(* Logix 5000 AddOnInstructionDefinition export YAI_Assy_170_115_EIP_Hz; software revision 21.03 *)

ADD_ON_INSTRUCTION YAI_Assy_170_115_EIP_Hz   (* revision 1.0, vendor Yaskawa America, Inc. *)
// YAI Assembly 170 and 115
// Help:
// This add-on instruction is for use with input assemblie 166 and output assemblies 116.
// Node_Input_Assy is defined as the node's input assembly integer array.
// Node_Output_Assy is defined as the node's output assembly integer array.
// Torque limit/reference, torque compensation and torque output variables are only available with A1000.
VAR_IN_OUT
   Node_Input_Assy : AB:ETHERNET_MODULE_INT_24Bytes:I:0; {required}   // Input assembly words
   Node_Output_Assy : AB:ETHERNET_MODULE_INT_40Bytes:O:0; {required}   // Output assembly words
END_VAR
VAR_INPUT
   RunFwd : BOOL; {visible}   // Forward run command
   RunRev : BOOL; {visible}   // Reverse run command
   MFI_3 : BOOL; {visible}   // Multi-function input 3
   MFI_4 : BOOL; {visible}   // Multi-function input 4
   MFI_5 : BOOL; {visible}   // Multi-function input 5
   MFI_6 : BOOL; {visible}   // Multi-function input 6
   MFI_7 : BOOL; {visible}   // Multi-function input 7
   MFI_8 : BOOL; {visible}   // Multi-function input 8
   External_Fault : BOOL;   // External fault command (EF0)
   FaultReset : BOOL; {visible}   // Fault reset command
   MFO_1 : BOOL; {visible}   // Multi-function output (M1-M2 for A/P1000, MA/MB/MC for V1000)
   MFO_2 : BOOL; {visible}   // Multi-function output (M3-M4 for A/P1000, P1 for V1000)
   MFO_3 : BOOL; {visible}   // Multi-function output (M5-M6 for A/P1000, P2 for V1000)
   Freq_Ref : REAL; {visible}   // Frequency reference command in Hz (xx.xx resolution)
   Torq_Ref_Limit : REAL; {visible}   // Torque reference/limit (A1000 only)
   Torq_Comp : REAL; {visible}   // Torque compensation command (A1000 only)
   Analog_Output_1 : REAL;   // Analog output 1 level command
   Analog_Output_2 : REAL;   // Analog output 2 level command
   Digital_Output_1 : BOOL;   // Digital output 1 activation - M1-M2
   Digital_Output_2 : BOOL;   // Digital output 2 activation - M3-M4
   Digital_Output_3 : BOOL;   // Digital output 3 activation - M5-M6
   Digital_Output_Fault_Enable : BOOL;   // Bit to enable control of fault output relay over the network
   Digital_Output_Fault : BOOL;   // Fault relay activation - MA-MB-MC
END_VAR
VAR_OUTPUT
   Running : BOOL; {access Read Only, visible}   // Drive running forward status bit
   ZSP : BOOL; {access Read Only, visible}   // Drive zero speed status bit
   RunningRev : BOOL; {access Read Only, visible}   // Drive running reverse status bit
   Reset : BOOL; {access Read Only, visible}   // Drive reset command status bit
   At_Speed : BOOL; {access Read Only, visible}   // Drive at commanded speed status bit
   Ready : BOOL; {access Read Only, visible}   // Drive ready status bit
   Alarm : BOOL; {access Read Only, visible}   // Drive alarm status bit
   Faulted : BOOL; {access Read Only, visible}   // Drive faulted status bit
   OPE : BOOL; {access Read Only}   // OPE alarm/fault present
   UV : BOOL; {access Read Only}   // Drive in UV (undervoltage) state status bit
   NetCtrlStatus : BOOL; {access Read Only, visible}   // Drive network run source status bit (1 = source coming from network)
   MFO_1_Status : BOOL; {access Read Only, visible}   // Drive multi-function output 1 (M1-M2 for A/P1000, MA/MB/MC for V1000) status
   MFO_2_Status : BOOL; {access Read Only, visible}   // Drive multi-function output 1 (M3-M4 for A/P1000, P1 for V1000) status
   MFO_3_Status : BOOL; {access Read Only, visible}   // Drive multi-function output 1 (M5-M6 for A/P1000, P2 for V1000) status
   ZSV : BOOL; {access Read Only, visible}   // Drive zero servo completed status bit
   Motor_Speed : REAL; {access Read Only, visible}   // Motor speed in Hz (xx.xx resolution)
   Custom_In_1 : INT; {access Read Only}
   Custom_In_2 : INT; {access Read Only}
   Custom_In_3 : INT; {access Read Only}
   Custom_In_4 : INT; {access Read Only}
   Custom_In_5 : INT; {access Read Only}
   Custom_In_6 : INT; {access Read Only}
   Custom_In_7 : INT; {access Read Only}
   Custom_In_8 : INT; {access Read Only}
   Custom_In_9 : INT; {access Read Only}
   Custom_In_10 : INT; {access Read Only}
END_VAR
VAR
   FRef_Convert : DINT;
   FOut_Convert : REAL;
   FOut_Temp : REAL;
   TRef_Convert : INT;
   TComp_Convert : INT;
   TOut_Convert : REAL;
   TOut_Temp : REAL;
   IOut_Temp : REAL;
   IOut_Convert : REAL;
   AO1_Convert : INT;
   AO2_Convert : INT;
   Motor_Speed_Temp : REAL;
   Motor_Speed_Convert : REAL;
   Freq_Cmd_Temp : REAL;
   Freq_Cmd_Convert : REAL;
   AI1_Temp : REAL;
   AI1_Convert : REAL;
   AI2_Temp : REAL; {access None}
   AI2_Convert : REAL; {access None}
   AI3_Temp : REAL; {access None}
   AI3_Convert : REAL; {access None}
END_VAR

ROUTINE Logic   (* ladder *)
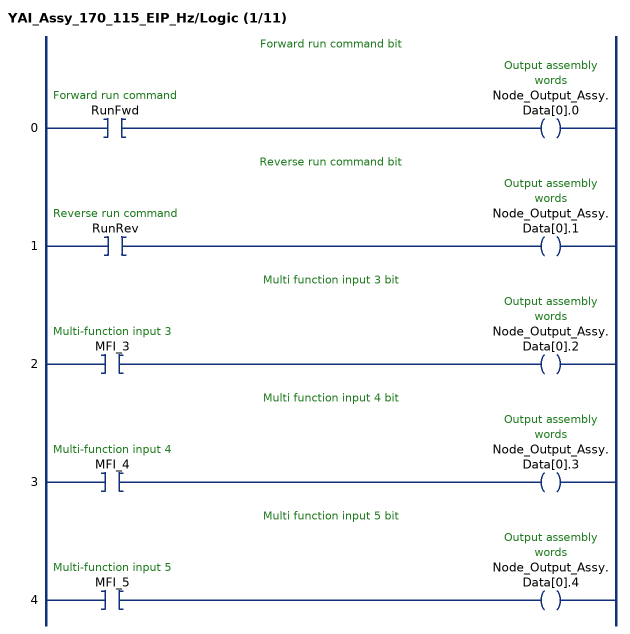
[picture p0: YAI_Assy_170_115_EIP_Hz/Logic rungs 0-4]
   // Forward run command bit
   0: XIC(RunFwd)OTE(Node_Output_Assy.Data[0].0);
   // Reverse run command bit
   1: XIC(RunRev)OTE(Node_Output_Assy.Data[0].1);
   // Multi function input 3 bit
   2: XIC(MFI_3)OTE(Node_Output_Assy.Data[0].2);
   // Multi function input 4 bit
   3: XIC(MFI_4)OTE(Node_Output_Assy.Data[0].3);
   // Multi function input 5 bit
   4: XIC(MFI_5)OTE(Node_Output_Assy.Data[0].4);
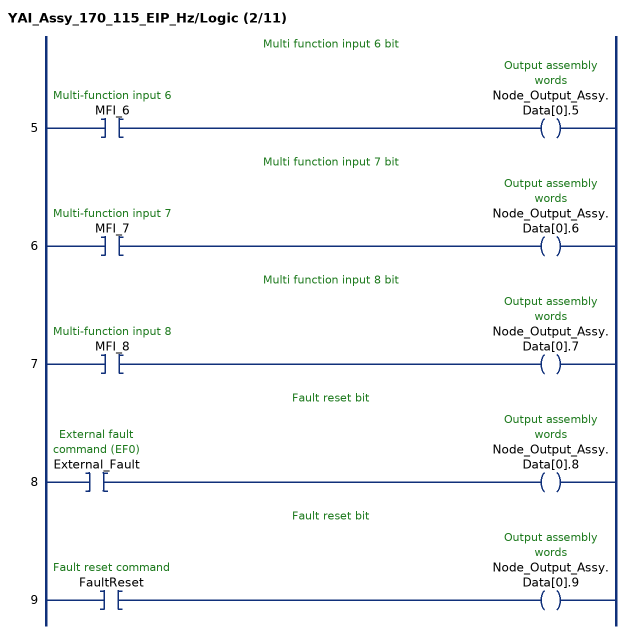
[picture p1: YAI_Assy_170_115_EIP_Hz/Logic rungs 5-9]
   // Multi function input 6 bit
   5: XIC(MFI_6)OTE(Node_Output_Assy.Data[0].5);
   // Multi function input 7 bit
   6: XIC(MFI_7)OTE(Node_Output_Assy.Data[0].6);
   // Multi function input 8 bit
   7: XIC(MFI_8)OTE(Node_Output_Assy.Data[0].7);
   // Fault reset bit
   8: XIC(External_Fault)OTE(Node_Output_Assy.Data[0].8);
   // Fault reset bit
   9: XIC(FaultReset)OTE(Node_Output_Assy.Data[0].9);
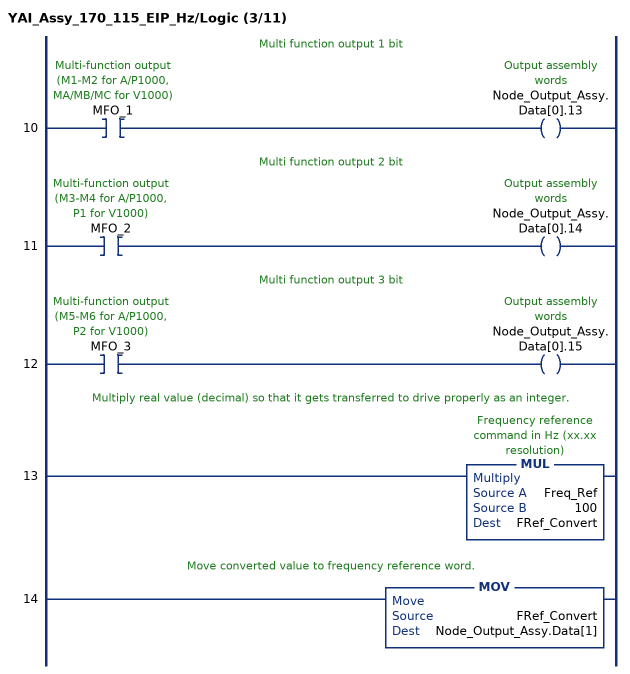
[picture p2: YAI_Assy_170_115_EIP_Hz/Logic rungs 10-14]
   // Multi function output 1 bit
   10: XIC(MFO_1)OTE(Node_Output_Assy.Data[0].13);
   // Multi function output 2 bit
   11: XIC(MFO_2)OTE(Node_Output_Assy.Data[0].14);
   // Multi function output 3 bit
   12: XIC(MFO_3)OTE(Node_Output_Assy.Data[0].15);
   // Multiply real value (decimal) so that it gets transferred to drive properly as an integer.
   13: MUL(Freq_Ref,100,FRef_Convert);
   // Move converted value to frequency reference word.
   14: MOV(FRef_Convert,Node_Output_Assy.Data[1]);
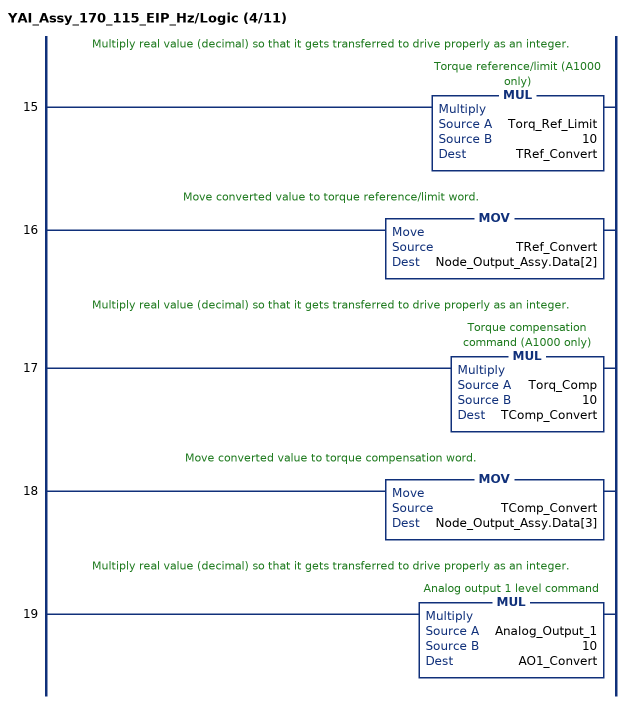
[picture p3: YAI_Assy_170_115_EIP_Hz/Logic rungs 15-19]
   // Multiply real value (decimal) so that it gets transferred to drive properly as an integer.
   15: MUL(Torq_Ref_Limit,10,TRef_Convert);
   // Move converted value to torque reference/limit word.
   16: MOV(TRef_Convert,Node_Output_Assy.Data[2]);
   // Multiply real value (decimal) so that it gets transferred to drive properly as an integer.
   17: MUL(Torq_Comp,10,TComp_Convert);
   // Move converted value to torque compensation word.
   18: MOV(TComp_Convert,Node_Output_Assy.Data[3]);
   // Multiply real value (decimal) so that it gets transferred to drive properly as an integer.
   19: MUL(Analog_Output_1,10,AO1_Convert);
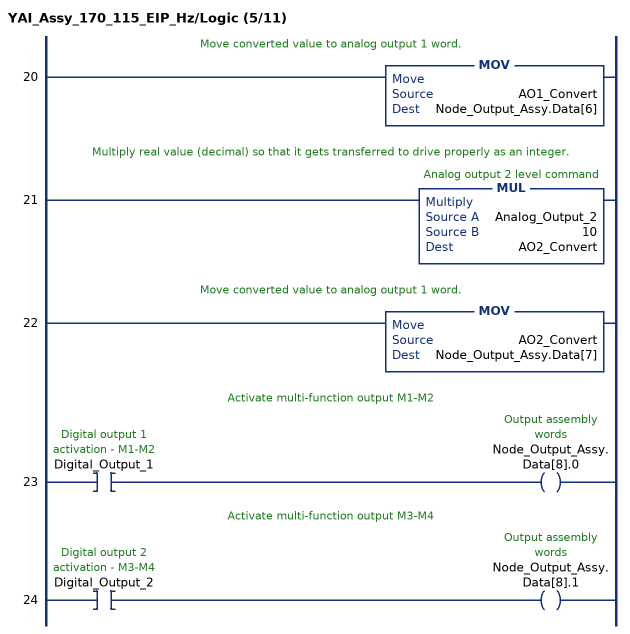
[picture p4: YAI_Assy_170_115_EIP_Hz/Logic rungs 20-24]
   // Move converted value to analog output 1 word.
   20: MOV(AO1_Convert,Node_Output_Assy.Data[6]);
   // Multiply real value (decimal) so that it gets transferred to drive properly as an integer.
   21: MUL(Analog_Output_2,10,AO2_Convert);
   // Move converted value to analog output 1 word.
   22: MOV(AO2_Convert,Node_Output_Assy.Data[7]);
   // Activate multi-function output M1-M2
   23: XIC(Digital_Output_1)OTE(Node_Output_Assy.Data[8].0);
   // Activate multi-function output M3-M4
   24: XIC(Digital_Output_2)OTE(Node_Output_Assy.Data[8].1);
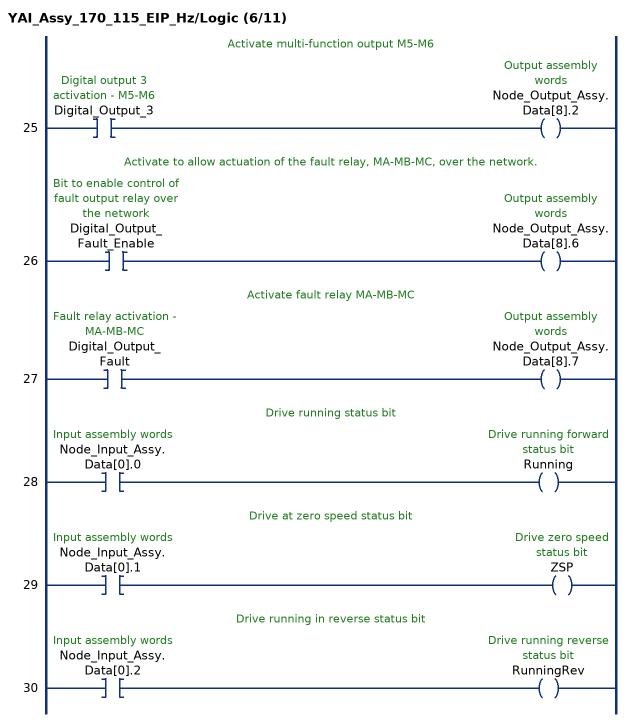
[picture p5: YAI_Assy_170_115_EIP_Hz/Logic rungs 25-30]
   // Activate multi-function output M5-M6
   25: XIC(Digital_Output_3)OTE(Node_Output_Assy.Data[8].2);
   // Activate to allow actuation of the fault relay, MA-MB-MC, over the network.
   26: XIC(Digital_Output_Fault_Enable)OTE(Node_Output_Assy.Data[8].6);
   // Activate fault relay MA-MB-MC
   27: XIC(Digital_Output_Fault)OTE(Node_Output_Assy.Data[8].7);
   // Drive running status bit
   28: XIC(Node_Input_Assy.Data[0].0)OTE(Running);
   // Drive at zero speed status bit
   29: XIC(Node_Input_Assy.Data[0].1)OTE(ZSP);
   // Drive running in reverse status bit
   30: XIC(Node_Input_Assy.Data[0].2)OTE(RunningRev);
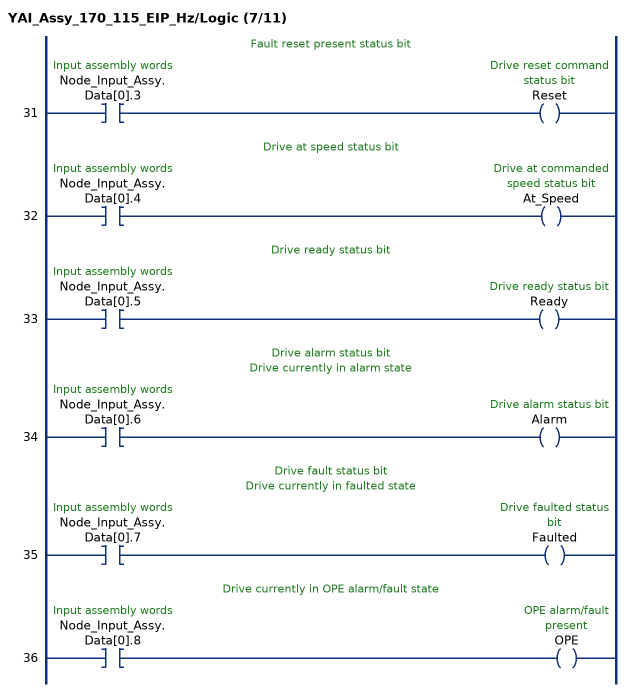
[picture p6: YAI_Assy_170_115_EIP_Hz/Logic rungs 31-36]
   // Fault reset present status bit
   31: XIC(Node_Input_Assy.Data[0].3)OTE(Reset);
   // Drive at speed status bit
   32: XIC(Node_Input_Assy.Data[0].4)OTE(At_Speed);
   // Drive ready status bit
   33: XIC(Node_Input_Assy.Data[0].5)OTE(Ready);
   // Drive alarm status bit
   // Drive currently in alarm state
   34: XIC(Node_Input_Assy.Data[0].6)OTE(Alarm);
   // Drive fault status bit
   // Drive currently in faulted state
   35: XIC(Node_Input_Assy.Data[0].7)OTE(Faulted);
   // Drive currently in OPE alarm/fault state
   36: XIC(Node_Input_Assy.Data[0].8)OTE(OPE);
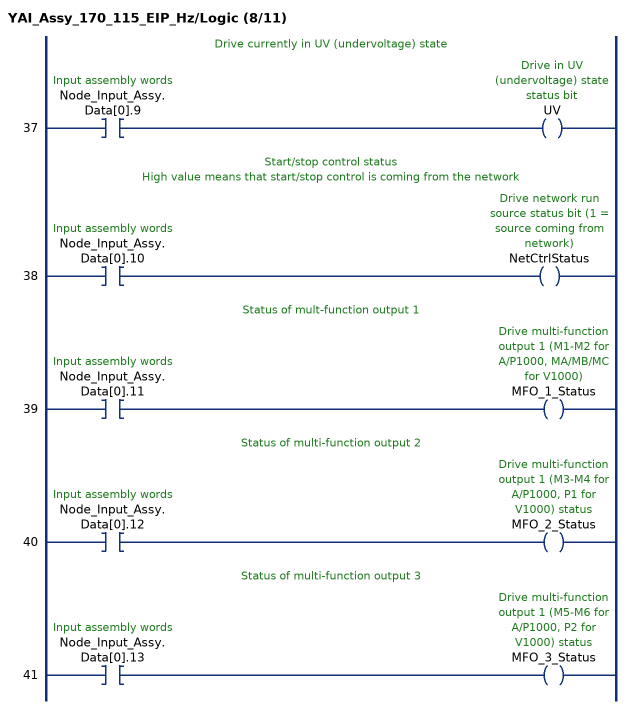
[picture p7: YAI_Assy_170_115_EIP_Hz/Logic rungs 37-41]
   // Drive currently in UV (undervoltage) state
   37: XIC(Node_Input_Assy.Data[0].9)OTE(UV);
   // Start/stop control status
   // High value means that start/stop control is coming from the network
   38: XIC(Node_Input_Assy.Data[0].10)OTE(NetCtrlStatus);
   // Status of mult-function output 1
   39: XIC(Node_Input_Assy.Data[0].11)OTE(MFO_1_Status);
   // Status of multi-function output 2
   40: XIC(Node_Input_Assy.Data[0].12)OTE(MFO_2_Status);
   // Status of multi-function output 3
   41: XIC(Node_Input_Assy.Data[0].13)OTE(MFO_3_Status);
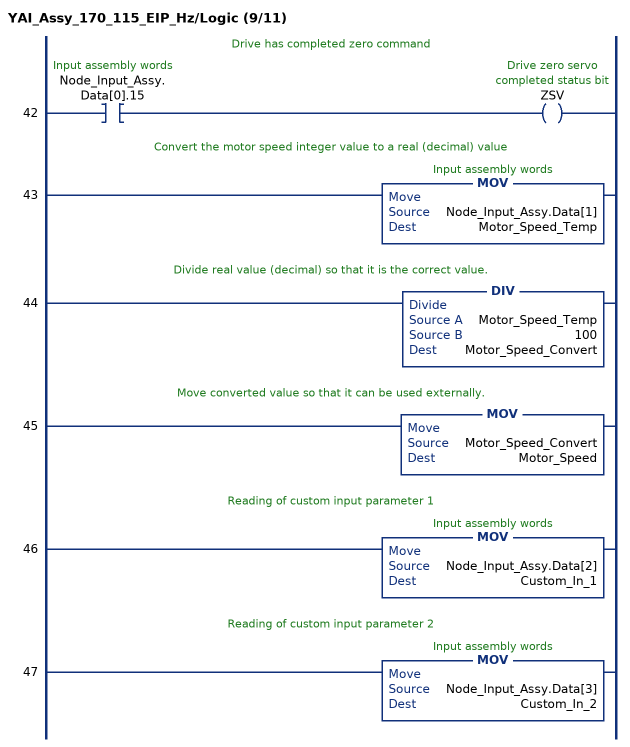
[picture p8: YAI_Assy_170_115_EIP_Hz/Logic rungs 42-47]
   // Drive has completed zero command
   42: XIC(Node_Input_Assy.Data[0].15)OTE(ZSV);
   // Convert the motor speed integer value to a real (decimal) value
   43: MOV(Node_Input_Assy.Data[1],Motor_Speed_Temp);
   // Divide real value (decimal) so that it is the correct value.
   44: DIV(Motor_Speed_Temp,100,Motor_Speed_Convert);
   // Move converted value so that it can be used externally.
   45: MOV(Motor_Speed_Convert,Motor_Speed);
   // Reading of custom input parameter 1
   46: MOV(Node_Input_Assy.Data[2],Custom_In_1);
   // Reading of custom input parameter 2
   47: MOV(Node_Input_Assy.Data[3],Custom_In_2);
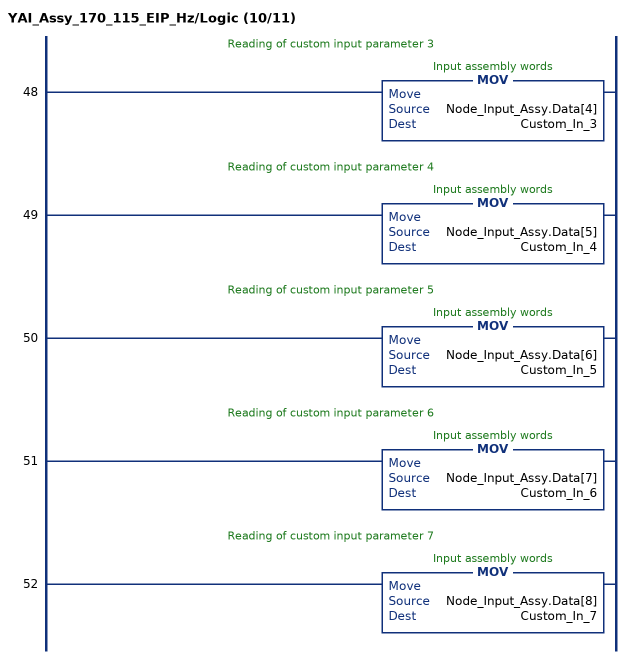
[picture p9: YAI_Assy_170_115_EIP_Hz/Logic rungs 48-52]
   // Reading of custom input parameter 3
   48: MOV(Node_Input_Assy.Data[4],Custom_In_3);
   // Reading of custom input parameter 4
   49: MOV(Node_Input_Assy.Data[5],Custom_In_4);
   // Reading of custom input parameter 5
   50: MOV(Node_Input_Assy.Data[6],Custom_In_5);
   // Reading of custom input parameter 6
   51: MOV(Node_Input_Assy.Data[7],Custom_In_6);
   // Reading of custom input parameter 7
   52: MOV(Node_Input_Assy.Data[8],Custom_In_7);
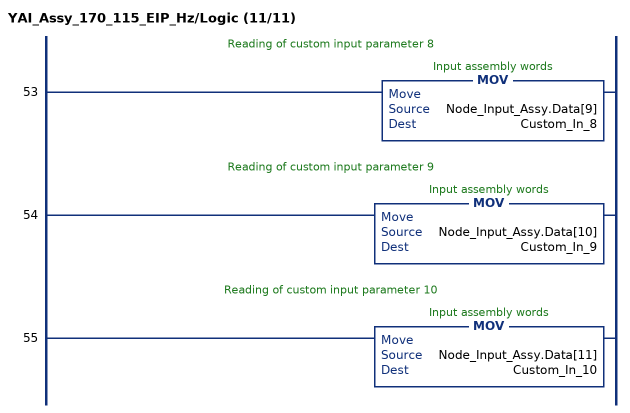
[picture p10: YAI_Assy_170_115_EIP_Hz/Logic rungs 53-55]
   // Reading of custom input parameter 8
   53: MOV(Node_Input_Assy.Data[9],Custom_In_8);
   // Reading of custom input parameter 9
   54: MOV(Node_Input_Assy.Data[10],Custom_In_9);
   // Reading of custom input parameter 10
   55: MOV(Node_Input_Assy.Data[11],Custom_In_10);
END_ROUTINE
END_ADD_ON_INSTRUCTION
